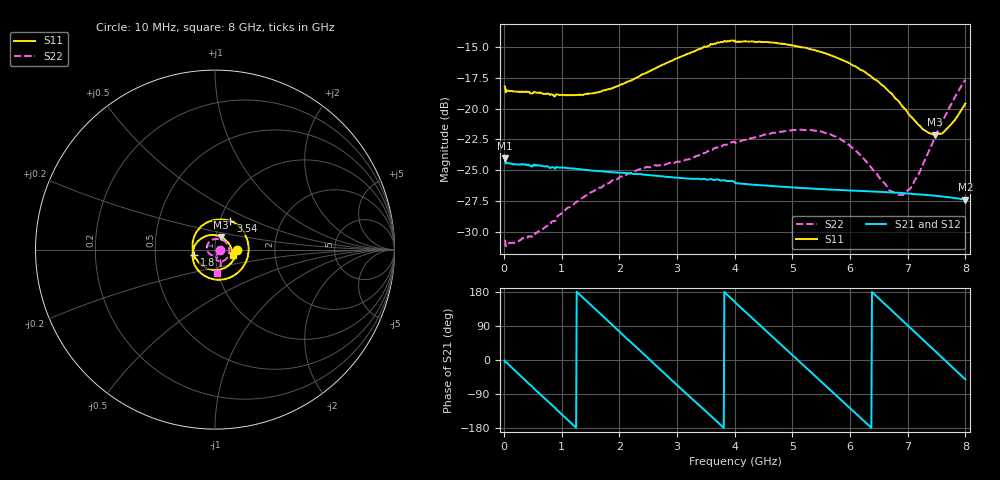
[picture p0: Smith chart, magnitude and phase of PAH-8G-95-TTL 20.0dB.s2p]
! MTS Systemtechnik GmbH
! S-Parameters
! Model: PAH-8G/95-TTL
! Attenuation Step: 20.0dB
! Rohde & Schwarz ZVB8 2Ports - Version 4.11 - 1145.1010k08 SN: 100119
! S2P File Measurements:
! S11 S21 S12 S22
# HZ  S  DB  R  50.00
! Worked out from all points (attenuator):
!   800 points, 10 MHz to 8 GHz, reference 50 ohm
!   highest |S21| = -24.02 dB at 10 MHz (marker M1); lowest = -27.4 dB at 8 GHz (marker M2)
!   lowest |S11| = -22.1 dB at 7.47 GHz (marker M3), VSWR 1.17, Z = 52.9 + j7.54 ohm
!   |S11| at or under -10 dB: start of sweep to end of sweep
!   |S22| runs from -31.2 to -17.6 dB; largest |S21 - S12| = 0.0009
!   S11 on the Smith chart (normalised r, x): 10 MHz: 1.28, -0.01; 1.8 GHz: 0.79, -0.05; 3.54 GHz: 1.12, +0.37; 8 GHz: 1.22, -0.08
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1e7  -18.19 -1.4  -24.02 -1.2  -23.94 -1.2  -30.67 -4.8
2e8  -18.61 -19.2  -24.52 -29.2  -24.52 -29.2  -30.88 -29.3
6.4e8  -18.71 -60.4  -24.63 -92.2  -24.62 -92.2  -29.87 -90.5
1.03e9  -18.88 -96.8  -24.79 -147.5  -24.80 -147.5  -28.40 -138.5
1.35e9  -18.89 -125.9  -24.94 167.1  -24.95 167.2  -27.30 -171.8
1.8e9  -18.43 -164.8  -25.13 103.3  -25.13 103.5  -26.08 148.5
2.3e9  -17.48 154.1  -25.32 33.0  -25.31 33.0  -25.00 112.9
2.68e9  -16.58 124.7  -25.48 -21.1  -25.48 -20.8  -24.62 91.3
3.11e9  -15.67 92.2  -25.65 -81.7  -25.66 -81.9  -24.23 69.3
3.54e9  -14.91 61.8  -25.77 -141.0  -25.76 -140.7  -23.45 51.7
4.01e9  -14.56 26.7  -26.05 151.7  -26.04 151.7  -22.79 30.5
4.63e9  -14.62 -17.6  -26.28 64.7  -26.28 64.7  -22.00 1.3
4.99e9  -14.84 -43.6  -26.40 14.4  -26.40 14.4  -21.74 -17.2
5.34e9  -15.19 -69.3  -26.50 -34.3  -26.50 -34.3  -21.75 -35.6
5.72e9  -15.76 -98.6  -26.59 -87.4  -26.61 -87.5  -22.22 -55.5
6.11e9  -16.60 -131.6  -26.68 -142.6  -26.69 -142.6  -23.46 -73.9
6.67e9  -18.59 174.5  -26.79 138.4  -26.79 138.4  -26.57 -83.4
6.88e9  -19.63 151.3  -26.85 108.5  -26.86 108.4  -27.02 -76.7
7.04e9  -20.58 130.9  -26.91 85.7  -26.91 85.7  -26.51 -69.5
7.47e9  -22.12 64.7  -27.08 24.5  -27.08 24.4  -22.33 -65.5
7.66e9  -21.72 32.6  -27.17 -2.6  -27.17 -2.7  -20.48 -70.9
8e9  -19.59 -17.6  -27.39 -51.3  -27.39 -51.3  -17.65 -86.0
